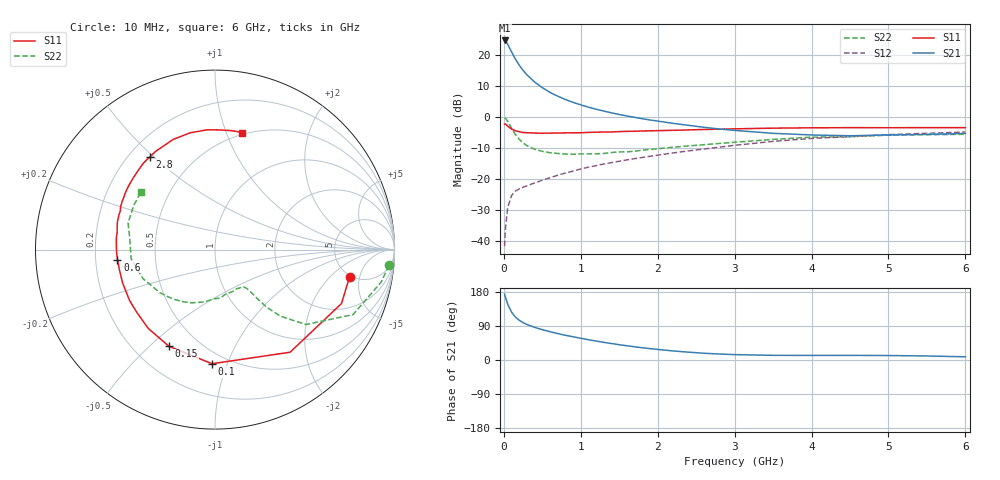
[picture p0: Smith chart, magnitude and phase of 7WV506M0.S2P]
! Infineon Technologies  Discrete & RF Semiconductors
! BFS17W
! Si NPN RF Bipolar Junction Transistor in SOT323
! VCE = 0.5 V  IC = 6 mA
! Common Emitter S-Parameters:  August  1999
# GHz  S  MA  R  50
!  f  S11  S21  S12  S22
! GHz  MAG  ANG  MAG  ANG  MAG  ANG  MAG  ANG
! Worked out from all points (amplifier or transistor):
!   36 points, 10 MHz to 6 GHz, reference 50 ohm
!   highest |S21| = 24.6 dB at 10 MHz (marker M1)
!   |S21| within 3 dB of that: start of sweep to 86.91 MHz
!   unconditionally stable (mu >= 1): 387.6 MHz to end of sweep
!   at 250 MHz: K = 0.74, MSG = 18.8 dB, |S12| = -22.7 dB
!   at 1.4 GHz: K = 1.44, MAG = 4.1 dB, |S12| = -14.7 dB
!   at 6 GHz: K = 1.15, MAG = -2.6 dB, |S12| = -4.9 dB
!   S11 on the Smith chart (normalised r, x): 10 MHz: 4.83, -3.55; 100 MHz: 0.41, -0.88; 150 MHz: 0.34, -0.58; 600 MHz: 0.29, -0.05; 2.8 GHz: 0.28, +0.49; 6 GHz: 0.48, +1.14
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0.01  0.765 -11.5  16.89 173.5  0.0083 82.0  0.9729 -5.2
0.02  0.7661 -23.1  16.7 166.0  0.0155 79.9  0.9432 -11.1
0.05  0.7085 -53.8  14.73 147.4  0.0348 64.7  0.8501 -25.2
0.1  0.6361 -91.5  11.11 126.4  0.0541 49.7  0.6564 -39.5
0.15  0.5967 -115.5  8.484 113.3  0.0639 43.4  0.5197 -45.5
0.2  0.5755 -130.3  6.763 104.9  0.0692 41.5  0.4357 -48.0
0.25  0.5587 -141.2  5.571 98.7  0.0734 40.4  0.3794 -48.9
0.3  0.5541 -149.2  4.73 93.8  0.0778 41.2  0.3443 -49.4
0.4  0.5473 -160.5  3.625 86.1  0.0862 42.9  0.2999 -50.0
0.5  0.5443 -168.3  2.939 80.0  0.0955 45.2  0.2785 -50.8
0.6  0.5462 -174.1  2.469 74.7  0.1047 47.1  0.2643 -52.3
0.7  0.5489 -178.9  2.146 69.8  0.115 48.7  0.257 -55.1
0.8  0.5505 176.6  1.899 65.3  0.1245 49.6  0.252 -58.4
1.1  0.5609 166.3  1.427 53.5  0.1549 51.4  0.2532 -69.2
1.3  0.5689 160.1  1.234 46.5  0.1741 51.7  0.2572 -78.0
1.6  0.583 152.5  1.03 37.6  0.2026 51.8  0.2734 -90.2
2.2  0.606 138.6  0.784 23.9  0.2622 50.7  0.324 -113.7
2.8  0.6316 125.2  0.637 15.8  0.3246 47.5  0.3726 -135.5
3.5  0.6565 110.8  0.542 12.3  0.402 41.5  0.4328 -158.0
4.5  0.669 93.7  0.495 12.2  0.4799 30.3  0.4787 172.6
5.5  0.6695 81.6  0.522 10.6  0.5427 20.7  0.5153 151.5
6  0.6694 76.8  0.539 8.4  0.5697 16.0  0.5225 141.9
